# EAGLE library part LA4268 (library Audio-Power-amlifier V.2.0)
The LA4268 is a SANYO 10 W power amplifier intended for televisions. This IC has a series of pin compatible monaural and 2- channel power amplifiers, thus allows the end product to use a common circuit boad.
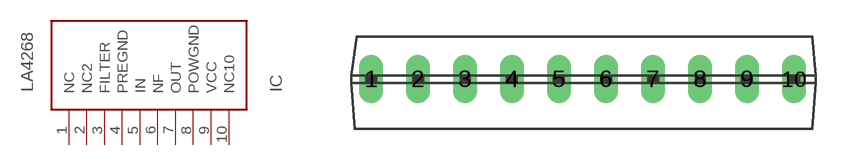
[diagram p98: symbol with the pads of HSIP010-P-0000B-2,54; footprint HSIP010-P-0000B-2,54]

Designator prefix IC

## LA42683248-SIP10HD  [HSIP010-P-0000B-2,54]
1  NC  nc
2  NC2  nc
3  FILTER
4  PREGND  pwr
5  IN  in
6  NF
7  OUT  out
8  POWGND  pwr
9  VCC  pwr
10  NC10  nc

## Footprint HSIP010-P-0000B-2,54 (pad centres in mm)
drill 0.8 long: 1 -11.43,0; 2 -8.89,0; 3 -6.35,0; 4 -3.81,0; 5 -1.27,0; 6 1.27,0; 7 3.81,0; 8 6.35,0; 9 8.89,0; 10 11.43,0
